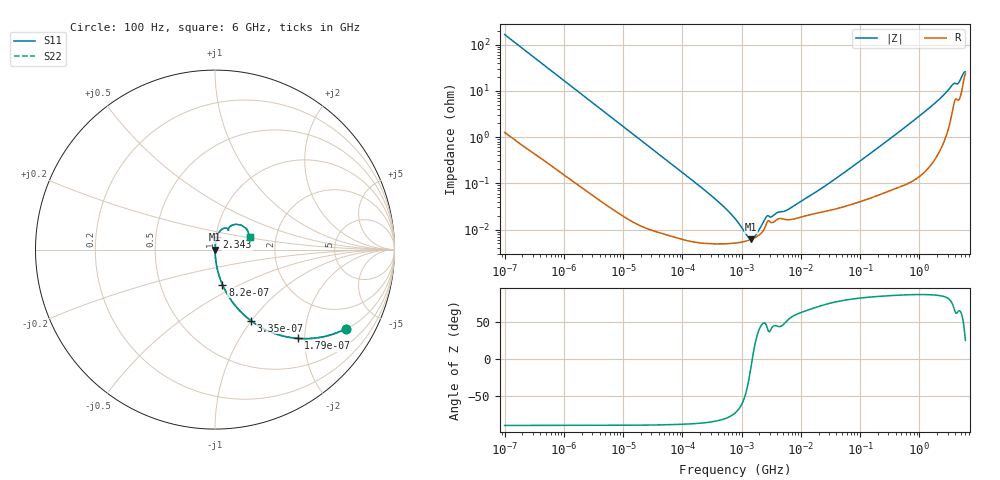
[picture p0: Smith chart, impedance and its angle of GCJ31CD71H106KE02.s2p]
!Murata Part Number: GCJ31CD71H106KE02
!These Parameters are Measured in Series Mode Connection
!Data Generated on Mar 13, 2026
!  o--ll--o
!Port1  Port2
!  o------o
!Operation Temp=25[degC], DC Bias Voltage=0[V]
!Freq. Start=100[Hz] Stop=6[GHz] 401[Steps]
# Hz S RI R 50
!Freq.(Hz) S11(Real) S11(Imag) S21(Real) S21(Imag) S12(Real) S12(Imag) S22(Real) S22(Imag)
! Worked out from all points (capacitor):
!   401 points, 100 Hz to 6 GHz, reference 50 ohm
!   read as one part in series: C = 9.62 uF near 109 Hz
!   lowest |Z| = 6.2 mohm at 1.45 MHz (marker M1)
!   series resonance near 1.517 MHz, so ESL is about 1.1 nH
!   S11 on the Smith chart (normalised r, x): 100 Hz: 1.03, -3.30; 179 Hz: 1.01, -1.85; 335 Hz: 1.01, -0.99; 820 Hz: 1.00, -0.41; 2.343 GHz: 1.01, +0.14; 6 GHz: 1.46, +0.22
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100  0.7302 -0.4401  0.2698 0.4401  0.2698 0.4401  0.7302 -0.4401
179  0.4617 -0.4946  0.5383 0.4946  0.5383 0.4946  0.4617 -0.4946
335  0.1995 -0.3955  0.8005 0.3955  0.8005 0.3955  0.1995 -0.3955
501  0.1015 -0.2977  0.8985 0.2977  0.8985 0.2977  0.1015 -0.2977
820  0.0414 -0.1948  0.9586 0.1948  0.9586 0.1948  0.0414 -0.1948
2008  0.00773 -0.0829  0.9923 0.0829  0.9923 0.0829  0.00773 -0.0829
6433  0.000971 -0.0262  0.999 0.0262  0.999 0.0262  0.000971 -0.0262
40335  0.000104 -0.00423  0.9999 0.00423  0.9999 0.00423  0.000104 -0.00423
316350  4.94e-05 -0.000522  1 0.000522  1 0.000522  4.94e-05 -0.000522
774597  5.09e-05 -0.000165  0.9999 0.000165  0.9999 0.000165  5.09e-05 -0.000165
1059725  5.43e-05 -8.39e-05  0.9999 8.39e-05  0.9999 8.39e-05  5.43e-05 -8.39e-05
1449809  6.11e-05 -1.04e-05  0.9999 1.04e-05  0.9999 1.04e-05  6.11e-05 -1.04e-05
1896632  7.3e-05 5.3e-05  0.9999 -5.3e-05  0.9999 -5.3e-05  7.3e-05 5.3e-05
2713602  0.000147 0.000134  0.9999 -0.000134  0.9999 -0.000134  0.000147 0.000134
5809218  0.000163 0.000206  0.9998 -0.000206  0.9998 -0.000206  0.000163 0.000206
1.555665e7  0.000214 0.000534  0.9998 -0.000534  0.9998 -0.000534  0.000214 0.000534
3.124326e8  0.000761 0.00894  0.9992 -0.00894  0.9992 -0.00894  0.000761 0.00894
2.34314e9  0.0107 0.0704  0.9893 -0.0704  0.9893 -0.0704  0.0107 0.0704
3.666503e9  0.0526 0.1198  0.9474 -0.1198  0.9474 -0.1198  0.0526 0.1198
4.586474e9  0.0735 0.1163  0.9265 -0.1163  0.9265 -0.1163  0.0735 0.1163
5.245841e9  0.1175 0.1413  0.8825 -0.1413  0.8825 -0.1413  0.1175 0.1413
6e9  0.1949 0.0719  0.8051 -0.0719  0.8051 -0.0719  0.1949 0.0719
